FUNCTION_BLOCK "IMAC_MOTOR1_CALL"
TITLE =Function calls for MOTOR1 objects
//Parameter Description for Function MOTOR1 (FB80):
//-------------------------------------------------
//OBJ:     Ascending Object number for MOTOR1 (1...x)
//
//RMOT:    'REMOTE'     Feedback
//                      0 = Local
//                      1 = Remote
//
//RUN:     'RUN'        Feedback
//                      0 = Stopped
//                      1 = Running
//
//FAUL     'EXT. FAULT' Feedback. Function depends on Mode Switch 'ExtFaultNC':
//                      If 'ExtFaultNC' = 0 :       0 = OK,    1 = Fault
//                      If 'ExtFaultNC' = 1 :       0 = Fault, 1 = OK
//
//BLKO:    'BLACKOUT'   Feedback
//                      0 = No Blackout
//                      1 = Blackout
//
//ACOM:    'AUTO' Mode  Command Interface (only active, if 'REMOTE'+'AUTO')
//                      Bit  0       : BlackoutStart
//                      Bit  1       : StandbyActive
//                      Bit  7       : FetchData Command
//                      Bit  8       : Start Command
//                      Bit  9       : Stop  Command
//                      Bit 10       : Failure input from Automatic Function
//                      Bit 11       : Lock 'Start / Stop'
//                      Bit 12       : Emergency Off Command
//
//PCONF:   (leave empty, refers to local instance data in Instance DB)
//
//MSTA:    'START'      Output to Motor
//                      0 = No Command
//                      1 = Start Command
//
//MSTO:    'STOP'       Output to Motor
//                      0 = No Command
//                      1 = Stop Command
//
//ASTAT:   'AUTO' Mode  Status Interface
//                      Bit  8       : Running
//                      Bit  9       : Local
//                      Bit 10       : Manual
//                      Bit 11       : Auto
//                      Bit 12       : Failure
//                      Bit 13       : BlackOut
//                      Bit 14       : Starting
//                      Bit 15       : Restarting
//
//OSSTAT:  OS Status Word
//                      Value = 0    : Undefined
//                      Value = 1    : Running
//                      Value = 2    : Stopped
//                      Value = 3    : Starting
//                      Value = 4    : StandBy
//                      Value = 5    : Blackout
//                      Value + 256  : Local Mode  (Offset Value)
//                      Value + 512  : Manual Mode (Offset Value)
//                      Value + 1024 : Auto Mode   (Offset Value)
//
//OSALARM: OS Alarm Word
//                      Value = 0    : Undefined
//                      Value = 1    : Normal
//                      Value = 2    : External Fault Alarm
//                      Value = 3    : Auto Failure Alarm
//                      Value = 4    : Action Alarm
//                      Value = 5    : Non-Feedback Alarm
//                      Value = 6    : Lock Start / Stop Commands
//                      Value = 7    : Emergency Off
//                      Value = 8    : Blackout
//
//OSCOM:   OS Command Interface
//                      Bit  0       : Start  Command
//                      Bit  1       : Stop   Command
//                      Bit  7       : Reset  Command
//                      Bit  9       : Manual Command
//                      Bit 10       : Auto   Command
AUTHOR : Hottendo
FAMILY : IMAC
VERSION : 0.2


VAR
  motorno_001 : "IMAC_MOTOR1";
  motorno_002 : "IMAC_MOTOR1";
  motorno_003 : "IMAC_MOTOR1";
  motorno_004 : "IMAC_MOTOR1";
  motorno_005 : "IMAC_MOTOR1";
  motorno_006 : "IMAC_MOTOR1";
  motorno_007 : "IMAC_MOTOR1";
  motorno_008 : "IMAC_MOTOR1";
  motorno_009 : "IMAC_MOTOR1";
  motorno_010 : "IMAC_MOTOR1";
  motorno_011 : "IMAC_MOTOR1";
  motorno_012 : "IMAC_MOTOR1";
  motorno_013 : "IMAC_MOTOR1";
  motorno_014 : "IMAC_MOTOR1";
  motorno_015 : "IMAC_MOTOR1";
  motorno_016 : "IMAC_MOTOR1";
  motorno_017 : "IMAC_MOTOR1";
  motorno_018 : "IMAC_MOTOR1";
  motorno_019 : "IMAC_MOTOR1";
  motorno_020 : "IMAC_MOTOR1";
  motorno_021 : "IMAC_MOTOR1";
  motorno_022 : "IMAC_MOTOR1";
  motorno_023 : "IMAC_MOTOR1";
  motorno_024 : "IMAC_MOTOR1";
  motorno_025 : "IMAC_MOTOR1";
  motorno_026 : "IMAC_MOTOR1";
  motorno_027 : "IMAC_MOTOR1";
  motorno_028 : "IMAC_MOTOR1";
  motorno_029 : "IMAC_MOTOR1";
  motorno_030 : "IMAC_MOTOR1";
  motorno_031 : "IMAC_MOTOR1";
  motorno_032 : "IMAC_MOTOR1";
  motorno_033 : "IMAC_MOTOR1";
  motorno_034 : "IMAC_MOTOR1";
  motorno_035 : "IMAC_MOTOR1";
  motorno_036 : "IMAC_MOTOR1";
  motorno_037 : "IMAC_MOTOR1";
  motorno_038 : "IMAC_MOTOR1";
  motorno_039 : "IMAC_MOTOR1";
  motorno_040 : "IMAC_MOTOR1";
  motorno_041 : "IMAC_MOTOR1";
  motorno_042 : "IMAC_MOTOR1";
  motorno_043 : "IMAC_MOTOR1";
  motorno_044 : "IMAC_MOTOR1";
  motorno_045 : "IMAC_MOTOR1";
  motorno_046 : "IMAC_MOTOR1";
  motorno_047 : "IMAC_MOTOR1";
  motorno_048 : "IMAC_MOTOR1";
  motorno_049 : "IMAC_MOTOR1";
  motorno_050 : "IMAC_MOTOR1";
END_VAR
BEGIN
NETWORK
TITLE =MOTOR1 Number 001

      CALL #motorno_001 (
           OBJ                      := 1,
           RMOT                     := E      2.0,
           RUN                      := E      2.1,
           FAUL                     := E      2.2,
           BLKO                     := E      2.3,
           ACOM                     := "IMAC_MOTOR1_I/O".MOTOR1_001_ACOM,
           MSTA                     := A      0.4,
           MSTO                     := A      0.5,
           ASTAT                    := "IMAC_MOTOR1_I/O".MOTOR1_001_ASTAT,
           OSSTAT                   := "IMAC_MOTOR1_I/O".MOTOR1_001_OSSTAT,
           OSALARM                  := "IMAC_MOTOR1_I/O".MOTOR1_001_OSALARM,
           OSCOM                    := "IMAC_MOTOR1_I/O".MOTOR1_001_OSCOM);

NETWORK
TITLE =MOTOR1 Number 002

      CALL #motorno_002 (
           OBJ                      := 2,
           RMOT                     := E      2.4,
           RUN                      := E      2.5,
           FAUL                     := E      2.6,
           BLKO                     := E      2.7,
           ACOM                     := "IMAC_MOTOR1_I/O".MOTOR1_002_ACOM,
           MSTA                     := A      0.6,
           MSTO                     := A      0.7,
           ASTAT                    := "IMAC_MOTOR1_I/O".MOTOR1_002_ASTAT,
           OSSTAT                   := "IMAC_MOTOR1_I/O".MOTOR1_002_OSSTAT,
           OSALARM                  := "IMAC_MOTOR1_I/O".MOTOR1_002_OSALARM,
           OSCOM                    := "IMAC_MOTOR1_I/O".MOTOR1_002_OSCOM);

NETWORK
TITLE =MOTOR1 Number 003

      CALL #motorno_003 (
           OBJ                      := 3,
           RMOT                     := E      3.0,
           RUN                      := E      3.1,
           FAUL                     := E      3.2,
           BLKO                     := E      3.3,
           ACOM                     := "IMAC_MOTOR1_I/O".MOTOR1_003_ACOM,
           MSTA                     := A      1.0,
           MSTO                     := A      1.1,
           ASTAT                    := "IMAC_MOTOR1_I/O".MOTOR1_003_ASTAT,
           OSSTAT                   := "IMAC_MOTOR1_I/O".MOTOR1_003_OSSTAT,
           OSALARM                  := "IMAC_MOTOR1_I/O".MOTOR1_003_OSALARM,
           OSCOM                    := "IMAC_MOTOR1_I/O".MOTOR1_003_OSCOM);

NETWORK
TITLE =MOTOR1 Number 004

      CALL #motorno_004 (
           OBJ                      := 4,
           RMOT                     := E      3.4,
           RUN                      := E      3.5,
           FAUL                     := E      3.6,
           BLKO                     := E      3.7,
           ACOM                     := "IMAC_MOTOR1_I/O".MOTOR1_004_ACOM,
           MSTA                     := A      1.2,
           MSTO                     := A      1.3,
           ASTAT                    := "IMAC_MOTOR1_I/O".MOTOR1_004_ASTAT,
           OSSTAT                   := "IMAC_MOTOR1_I/O".MOTOR1_004_OSSTAT,
           OSALARM                  := "IMAC_MOTOR1_I/O".MOTOR1_004_OSALARM,
           OSCOM                    := "IMAC_MOTOR1_I/O".MOTOR1_004_OSCOM);

NETWORK
TITLE =MOTOR1 Number 005

      CALL #motorno_005 (
           OBJ                      := 5,
           RMOT                     := E      4.0,
           RUN                      := E      4.1,
           FAUL                     := E      4.2,
           BLKO                     := E      4.3,
           ACOM                     := "IMAC_MOTOR1_I/O".MOTOR1_005_ACOM,
           MSTA                     := A      1.4,
           MSTO                     := A      1.5,
           ASTAT                    := "IMAC_MOTOR1_I/O".MOTOR1_005_ASTAT,
           OSSTAT                   := "IMAC_MOTOR1_I/O".MOTOR1_005_OSSTAT,
           OSALARM                  := "IMAC_MOTOR1_I/O".MOTOR1_005_OSALARM,
           OSCOM                    := "IMAC_MOTOR1_I/O".MOTOR1_005_OSCOM);

NETWORK
TITLE =MOTOR1 Number 006

      CALL #motorno_006 (
           OBJ                      := 6,
           RMOT                     := E      4.4,
           RUN                      := E      4.5,
           FAUL                     := E      4.6,
           BLKO                     := E      4.7,
           ACOM                     := "IMAC_MOTOR1_I/O".MOTOR1_006_ACOM,
           MSTA                     := A      1.6,
           MSTO                     := A      1.7,
           ASTAT                    := "IMAC_MOTOR1_I/O".MOTOR1_006_ASTAT,
           OSSTAT                   := "IMAC_MOTOR1_I/O".MOTOR1_006_OSSTAT,
           OSALARM                  := "IMAC_MOTOR1_I/O".MOTOR1_006_OSALARM,
           OSCOM                    := "IMAC_MOTOR1_I/O".MOTOR1_006_OSCOM);

NETWORK
TITLE =MOTOR1 Number 007

//*********** END of function Processing ! *******************************************************************
      BEA   ; // Move this Instruction down to the next Network to add one object !
//************************************************************************************************************

      CALL #motorno_007 (
           OBJ                      := 7,
           ACOM                     := "IMAC_MOTOR1_I/O".MOTOR1_007_ACOM,
           ASTAT                    := "IMAC_MOTOR1_I/O".MOTOR1_007_ASTAT,
           OSSTAT                   := "IMAC_MOTOR1_I/O".MOTOR1_007_OSSTAT,
           OSALARM                  := "IMAC_MOTOR1_I/O".MOTOR1_007_OSALARM,
           OSCOM                    := "IMAC_MOTOR1_I/O".MOTOR1_007_OSCOM);

NETWORK
TITLE =MOTOR1 Number 008

      CALL #motorno_008 (
           OBJ                      := 8,
           ACOM                     := "IMAC_MOTOR1_I/O".MOTOR1_008_ACOM,
           ASTAT                    := "IMAC_MOTOR1_I/O".MOTOR1_008_ASTAT,
           OSSTAT                   := "IMAC_MOTOR1_I/O".MOTOR1_008_OSSTAT,
           OSALARM                  := "IMAC_MOTOR1_I/O".MOTOR1_008_OSALARM,
           OSCOM                    := "IMAC_MOTOR1_I/O".MOTOR1_008_OSCOM);

NETWORK
TITLE =MOTOR1 Number 009

      CALL #motorno_009 (
           OBJ                      := 9,
           ACOM                     := "IMAC_MOTOR1_I/O".MOTOR1_009_ACOM,
           ASTAT                    := "IMAC_MOTOR1_I/O".MOTOR1_009_ASTAT,
           OSSTAT                   := "IMAC_MOTOR1_I/O".MOTOR1_009_OSSTAT,
           OSALARM                  := "IMAC_MOTOR1_I/O".MOTOR1_009_OSALARM,
           OSCOM                    := "IMAC_MOTOR1_I/O".MOTOR1_009_OSCOM);

NETWORK
TITLE =MOTOR1 Number 010

      CALL #motorno_010 (
           OBJ                      := 10,
           ACOM                     := "IMAC_MOTOR1_I/O".MOTOR1_010_ACOM,
           ASTAT                    := "IMAC_MOTOR1_I/O".MOTOR1_010_ASTAT,
           OSSTAT                   := "IMAC_MOTOR1_I/O".MOTOR1_010_OSSTAT,
           OSALARM                  := "IMAC_MOTOR1_I/O".MOTOR1_010_OSALARM,
           OSCOM                    := "IMAC_MOTOR1_I/O".MOTOR1_010_OSCOM);

NETWORK
TITLE =MOTOR1 Number 011

      CALL #motorno_011 (
           OBJ                      := 11,
           ACOM                     := "IMAC_MOTOR1_I/O".MOTOR1_011_ACOM,
           ASTAT                    := "IMAC_MOTOR1_I/O".MOTOR1_011_ASTAT,
           OSSTAT                   := "IMAC_MOTOR1_I/O".MOTOR1_011_OSSTAT,
           OSALARM                  := "IMAC_MOTOR1_I/O".MOTOR1_011_OSALARM,
           OSCOM                    := "IMAC_MOTOR1_I/O".MOTOR1_011_OSCOM);

NETWORK
TITLE =MOTOR1 Number 012

      CALL #motorno_012 (
           OBJ                      := 12,
           ACOM                     := "IMAC_MOTOR1_I/O".MOTOR1_012_ACOM,
           ASTAT                    := "IMAC_MOTOR1_I/O".MOTOR1_012_ASTAT,
           OSSTAT                   := "IMAC_MOTOR1_I/O".MOTOR1_012_OSSTAT,
           OSALARM                  := "IMAC_MOTOR1_I/O".MOTOR1_012_OSALARM,
           OSCOM                    := "IMAC_MOTOR1_I/O".MOTOR1_012_OSCOM);

NETWORK
TITLE =MOTOR1 Number 013

      CALL #motorno_013 (
           OBJ                      := 13,
           ACOM                     := "IMAC_MOTOR1_I/O".MOTOR1_013_ACOM,
           ASTAT                    := "IMAC_MOTOR1_I/O".MOTOR1_013_ASTAT,
           OSSTAT                   := "IMAC_MOTOR1_I/O".MOTOR1_013_OSSTAT,
           OSALARM                  := "IMAC_MOTOR1_I/O".MOTOR1_013_OSALARM,
           OSCOM                    := "IMAC_MOTOR1_I/O".MOTOR1_013_OSCOM);

NETWORK
TITLE =MOTOR1 Number 014

      CALL #motorno_014 (
           OBJ                      := 14,
           ACOM                     := "IMAC_MOTOR1_I/O".MOTOR1_014_ACOM,
           ASTAT                    := "IMAC_MOTOR1_I/O".MOTOR1_014_ASTAT,
           OSSTAT                   := "IMAC_MOTOR1_I/O".MOTOR1_014_OSSTAT,
           OSALARM                  := "IMAC_MOTOR1_I/O".MOTOR1_014_OSALARM,
           OSCOM                    := "IMAC_MOTOR1_I/O".MOTOR1_014_OSCOM);

NETWORK
TITLE =MOTOR1 Number 015

      CALL #motorno_015 (
           OBJ                      := 15,
           ACOM                     := "IMAC_MOTOR1_I/O".MOTOR1_015_ACOM,
           ASTAT                    := "IMAC_MOTOR1_I/O".MOTOR1_015_ASTAT,
           OSSTAT                   := "IMAC_MOTOR1_I/O".MOTOR1_015_OSSTAT,
           OSALARM                  := "IMAC_MOTOR1_I/O".MOTOR1_015_OSALARM,
           OSCOM                    := "IMAC_MOTOR1_I/O".MOTOR1_015_OSCOM);

NETWORK
TITLE =MOTOR1 Number 016

      CALL #motorno_016 (
           OBJ                      := 16,
           ACOM                     := "IMAC_MOTOR1_I/O".MOTOR1_016_ACOM,
           ASTAT                    := "IMAC_MOTOR1_I/O".MOTOR1_016_ASTAT,
           OSSTAT                   := "IMAC_MOTOR1_I/O".MOTOR1_016_OSSTAT,
           OSALARM                  := "IMAC_MOTOR1_I/O".MOTOR1_016_OSALARM,
           OSCOM                    := "IMAC_MOTOR1_I/O".MOTOR1_016_OSCOM);

NETWORK
TITLE =MOTOR1 Number 017

      CALL #motorno_017 (
           OBJ                      := 17,
           ACOM                     := "IMAC_MOTOR1_I/O".MOTOR1_017_ACOM,
           ASTAT                    := "IMAC_MOTOR1_I/O".MOTOR1_017_ASTAT,
           OSSTAT                   := "IMAC_MOTOR1_I/O".MOTOR1_017_OSSTAT,
           OSALARM                  := "IMAC_MOTOR1_I/O".MOTOR1_017_OSALARM,
           OSCOM                    := "IMAC_MOTOR1_I/O".MOTOR1_017_OSCOM);

NETWORK
TITLE =MOTOR1 Number 018

      CALL #motorno_018 (
           OBJ                      := 18,
           ACOM                     := "IMAC_MOTOR1_I/O".MOTOR1_018_ACOM,
           ASTAT                    := "IMAC_MOTOR1_I/O".MOTOR1_018_ASTAT,
           OSSTAT                   := "IMAC_MOTOR1_I/O".MOTOR1_018_OSSTAT,
           OSALARM                  := "IMAC_MOTOR1_I/O".MOTOR1_018_OSALARM,
           OSCOM                    := "IMAC_MOTOR1_I/O".MOTOR1_018_OSCOM);

NETWORK
TITLE =MOTOR1 Number 019

      CALL #motorno_019 (
           OBJ                      := 19,
           ACOM                     := "IMAC_MOTOR1_I/O".MOTOR1_019_ACOM,
           ASTAT                    := "IMAC_MOTOR1_I/O".MOTOR1_019_ASTAT,
           OSSTAT                   := "IMAC_MOTOR1_I/O".MOTOR1_019_OSSTAT,
           OSALARM                  := "IMAC_MOTOR1_I/O".MOTOR1_019_OSALARM,
           OSCOM                    := "IMAC_MOTOR1_I/O".MOTOR1_019_OSCOM);

NETWORK
TITLE =MOTOR1 Number 020

      CALL #motorno_020 (
           OBJ                      := 20,
           ACOM                     := "IMAC_MOTOR1_I/O".MOTOR1_020_ACOM,
           ASTAT                    := "IMAC_MOTOR1_I/O".MOTOR1_020_ASTAT,
           OSSTAT                   := "IMAC_MOTOR1_I/O".MOTOR1_020_OSSTAT,
           OSALARM                  := "IMAC_MOTOR1_I/O".MOTOR1_020_OSALARM,
           OSCOM                    := "IMAC_MOTOR1_I/O".MOTOR1_020_OSCOM);

NETWORK
TITLE =MOTOR1 Number 021

      CALL #motorno_021 (
           OBJ                      := 21,
           ACOM                     := "IMAC_MOTOR1_I/O".MOTOR1_021_ACOM,
           ASTAT                    := "IMAC_MOTOR1_I/O".MOTOR1_021_ASTAT,
           OSSTAT                   := "IMAC_MOTOR1_I/O".MOTOR1_021_OSSTAT,
           OSALARM                  := "IMAC_MOTOR1_I/O".MOTOR1_021_OSALARM,
           OSCOM                    := "IMAC_MOTOR1_I/O".MOTOR1_021_OSCOM);

NETWORK
TITLE =MOTOR1 Number 022

      CALL #motorno_022 (
           OBJ                      := 22,
           ACOM                     := "IMAC_MOTOR1_I/O".MOTOR1_022_ACOM,
           ASTAT                    := "IMAC_MOTOR1_I/O".MOTOR1_022_ASTAT,
           OSSTAT                   := "IMAC_MOTOR1_I/O".MOTOR1_022_OSSTAT,
           OSALARM                  := "IMAC_MOTOR1_I/O".MOTOR1_022_OSALARM,
           OSCOM                    := "IMAC_MOTOR1_I/O".MOTOR1_003_OSCOM);

NETWORK
TITLE =MOTOR1 Number 023

      CALL #motorno_023 (
           OBJ                      := 23,
           ACOM                     := "IMAC_MOTOR1_I/O".MOTOR1_023_ACOM,
           ASTAT                    := "IMAC_MOTOR1_I/O".MOTOR1_023_ASTAT,
           OSSTAT                   := "IMAC_MOTOR1_I/O".MOTOR1_023_OSSTAT,
           OSALARM                  := "IMAC_MOTOR1_I/O".MOTOR1_023_OSALARM,
           OSCOM                    := "IMAC_MOTOR1_I/O".MOTOR1_023_OSCOM);

NETWORK
TITLE =MOTOR1 Number 024

      CALL #motorno_024 (
           OBJ                      := 24,
           ACOM                     := "IMAC_MOTOR1_I/O".MOTOR1_024_ACOM,
           ASTAT                    := "IMAC_MOTOR1_I/O".MOTOR1_024_ASTAT,
           OSSTAT                   := "IMAC_MOTOR1_I/O".MOTOR1_024_OSSTAT,
           OSALARM                  := "IMAC_MOTOR1_I/O".MOTOR1_024_OSALARM,
           OSCOM                    := "IMAC_MOTOR1_I/O".MOTOR1_024_OSCOM);

NETWORK
TITLE =MOTOR1 Number 025

      CALL #motorno_025 (
           OBJ                      := 25,
           ACOM                     := "IMAC_MOTOR1_I/O".MOTOR1_025_ACOM,
           ASTAT                    := "IMAC_MOTOR1_I/O".MOTOR1_025_ASTAT,
           OSSTAT                   := "IMAC_MOTOR1_I/O".MOTOR1_025_OSSTAT,
           OSALARM                  := "IMAC_MOTOR1_I/O".MOTOR1_025_OSALARM,
           OSCOM                    := "IMAC_MOTOR1_I/O".MOTOR1_025_OSCOM);

NETWORK
TITLE =MOTOR1 Number 026

      CALL #motorno_026 (
           OBJ                      := 26,
           ACOM                     := "IMAC_MOTOR1_I/O".MOTOR1_026_ACOM,
           ASTAT                    := "IMAC_MOTOR1_I/O".MOTOR1_026_ASTAT,
           OSSTAT                   := "IMAC_MOTOR1_I/O".MOTOR1_026_OSSTAT,
           OSALARM                  := "IMAC_MOTOR1_I/O".MOTOR1_026_OSALARM,
           OSCOM                    := "IMAC_MOTOR1_I/O".MOTOR1_026_OSCOM);

NETWORK
TITLE =MOTOR1 Number 027

      CALL #motorno_027 (
           OBJ                      := 27,
           ACOM                     := "IMAC_MOTOR1_I/O".MOTOR1_027_ACOM,
           ASTAT                    := "IMAC_MOTOR1_I/O".MOTOR1_027_ASTAT,
           OSSTAT                   := "IMAC_MOTOR1_I/O".MOTOR1_027_OSSTAT,
           OSALARM                  := "IMAC_MOTOR1_I/O".MOTOR1_027_OSALARM,
           OSCOM                    := "IMAC_MOTOR1_I/O".MOTOR1_027_OSCOM);

NETWORK
TITLE =MOTOR1 Number 028

      CALL #motorno_028 (
           OBJ                      := 28,
           ACOM                     := "IMAC_MOTOR1_I/O".MOTOR1_028_ACOM,
           ASTAT                    := "IMAC_MOTOR1_I/O".MOTOR1_028_ASTAT,
           OSSTAT                   := "IMAC_MOTOR1_I/O".MOTOR1_028_OSSTAT,
           OSALARM                  := "IMAC_MOTOR1_I/O".MOTOR1_028_OSALARM,
           OSCOM                    := "IMAC_MOTOR1_I/O".MOTOR1_028_OSCOM);

NETWORK
TITLE =MOTOR1 Number 029

      CALL #motorno_029 (
           OBJ                      := 29,
           ACOM                     := "IMAC_MOTOR1_I/O".MOTOR1_029_ACOM,
           ASTAT                    := "IMAC_MOTOR1_I/O".MOTOR1_029_ASTAT,
           OSSTAT                   := "IMAC_MOTOR1_I/O".MOTOR1_029_OSSTAT,
           OSALARM                  := "IMAC_MOTOR1_I/O".MOTOR1_029_OSALARM,
           OSCOM                    := "IMAC_MOTOR1_I/O".MOTOR1_029_OSCOM);

NETWORK
TITLE =MOTOR1 Number 030

      CALL #motorno_030 (
           OBJ                      := 30,
           ACOM                     := "IMAC_MOTOR1_I/O".MOTOR1_030_ACOM,
           ASTAT                    := "IMAC_MOTOR1_I/O".MOTOR1_030_ASTAT,
           OSSTAT                   := "IMAC_MOTOR1_I/O".MOTOR1_030_OSSTAT,
           OSALARM                  := "IMAC_MOTOR1_I/O".MOTOR1_030_OSALARM,
           OSCOM                    := "IMAC_MOTOR1_I/O".MOTOR1_030_OSCOM);

NETWORK
TITLE =MOTOR1 Number 031

      CALL #motorno_031 (
           OBJ                      := 31,
           ACOM                     := "IMAC_MOTOR1_I/O".MOTOR1_031_ACOM,
           ASTAT                    := "IMAC_MOTOR1_I/O".MOTOR1_031_ASTAT,
           OSSTAT                   := "IMAC_MOTOR1_I/O".MOTOR1_031_OSSTAT,
           OSALARM                  := "IMAC_MOTOR1_I/O".MOTOR1_031_OSALARM,
           OSCOM                    := "IMAC_MOTOR1_I/O".MOTOR1_031_OSCOM);

NETWORK
TITLE =MOTOR1 Number 032

      CALL #motorno_032 (
           OBJ                      := 32,
           ACOM                     := "IMAC_MOTOR1_I/O".MOTOR1_032_ACOM,
           ASTAT                    := "IMAC_MOTOR1_I/O".MOTOR1_032_ASTAT,
           OSSTAT                   := "IMAC_MOTOR1_I/O".MOTOR1_032_OSSTAT,
           OSALARM                  := "IMAC_MOTOR1_I/O".MOTOR1_032_OSALARM,
           OSCOM                    := "IMAC_MOTOR1_I/O".MOTOR1_032_OSCOM);

NETWORK
TITLE =MOTOR1 Number 033

      CALL #motorno_033 (
           OBJ                      := 33,
           ACOM                     := "IMAC_MOTOR1_I/O".MOTOR1_033_ACOM,
           ASTAT                    := "IMAC_MOTOR1_I/O".MOTOR1_033_ASTAT,
           OSSTAT                   := "IMAC_MOTOR1_I/O".MOTOR1_033_OSSTAT,
           OSALARM                  := "IMAC_MOTOR1_I/O".MOTOR1_033_OSALARM,
           OSCOM                    := "IMAC_MOTOR1_I/O".MOTOR1_033_OSCOM);

NETWORK
TITLE =MOTOR1 Number 034

      CALL #motorno_034 (
           OBJ                      := 34,
           ACOM                     := "IMAC_MOTOR1_I/O".MOTOR1_034_ACOM,
           ASTAT                    := "IMAC_MOTOR1_I/O".MOTOR1_034_ASTAT,
           OSSTAT                   := "IMAC_MOTOR1_I/O".MOTOR1_034_OSSTAT,
           OSALARM                  := "IMAC_MOTOR1_I/O".MOTOR1_034_OSALARM,
           OSCOM                    := "IMAC_MOTOR1_I/O".MOTOR1_034_OSCOM);

NETWORK
TITLE =MOTOR1 Number 035

      CALL #motorno_035 (
           OBJ                      := 35,
           ACOM                     := "IMAC_MOTOR1_I/O".MOTOR1_035_ACOM,
           ASTAT                    := "IMAC_MOTOR1_I/O".MOTOR1_035_ASTAT,
           OSSTAT                   := "IMAC_MOTOR1_I/O".MOTOR1_035_OSSTAT,
           OSALARM                  := "IMAC_MOTOR1_I/O".MOTOR1_035_OSALARM,
           OSCOM                    := "IMAC_MOTOR1_I/O".MOTOR1_035_OSCOM);

NETWORK
TITLE =MOTOR1 Number 036

      CALL #motorno_036 (
           OBJ                      := 36,
           ACOM                     := "IMAC_MOTOR1_I/O".MOTOR1_036_ACOM,
           ASTAT                    := "IMAC_MOTOR1_I/O".MOTOR1_036_ASTAT,
           OSSTAT                   := "IMAC_MOTOR1_I/O".MOTOR1_036_OSSTAT,
           OSALARM                  := "IMAC_MOTOR1_I/O".MOTOR1_036_OSALARM,
           OSCOM                    := "IMAC_MOTOR1_I/O".MOTOR1_036_OSCOM);

NETWORK
TITLE =MOTOR1 Number 037

      CALL #motorno_037 (
           OBJ                      := 37,
           ACOM                     := "IMAC_MOTOR1_I/O".MOTOR1_037_ACOM,
           ASTAT                    := "IMAC_MOTOR1_I/O".MOTOR1_037_ASTAT,
           OSSTAT                   := "IMAC_MOTOR1_I/O".MOTOR1_037_OSSTAT,
           OSALARM                  := "IMAC_MOTOR1_I/O".MOTOR1_037_OSALARM,
           OSCOM                    := "IMAC_MOTOR1_I/O".MOTOR1_037_OSCOM);

NETWORK
TITLE =MOTOR1 Number 038

      CALL #motorno_038 (
           OBJ                      := 38,
           ACOM                     := "IMAC_MOTOR1_I/O".MOTOR1_038_ACOM,
           ASTAT                    := "IMAC_MOTOR1_I/O".MOTOR1_038_ASTAT,
           OSSTAT                   := "IMAC_MOTOR1_I/O".MOTOR1_038_OSSTAT,
           OSALARM                  := "IMAC_MOTOR1_I/O".MOTOR1_038_OSALARM,
           OSCOM                    := "IMAC_MOTOR1_I/O".MOTOR1_038_OSCOM);

NETWORK
TITLE =MOTOR1 Number 039

      CALL #motorno_039 (
           OBJ                      := 39,
           ACOM                     := "IMAC_MOTOR1_I/O".MOTOR1_039_ACOM,
           ASTAT                    := "IMAC_MOTOR1_I/O".MOTOR1_039_ASTAT,
           OSSTAT                   := "IMAC_MOTOR1_I/O".MOTOR1_039_OSSTAT,
           OSALARM                  := "IMAC_MOTOR1_I/O".MOTOR1_039_OSALARM,
           OSCOM                    := "IMAC_MOTOR1_I/O".MOTOR1_039_OSCOM);

NETWORK
TITLE =MOTOR1 Number 040

      CALL #motorno_040 (
           OBJ                      := 40,
           ACOM                     := "IMAC_MOTOR1_I/O".MOTOR1_040_ACOM,
           ASTAT                    := "IMAC_MOTOR1_I/O".MOTOR1_040_ASTAT,
           OSSTAT                   := "IMAC_MOTOR1_I/O".MOTOR1_040_OSSTAT,
           OSALARM                  := "IMAC_MOTOR1_I/O".MOTOR1_040_OSALARM,
           OSCOM                    := "IMAC_MOTOR1_I/O".MOTOR1_040_OSCOM);

NETWORK
TITLE =MOTOR1 Number 041

      CALL #motorno_041 (
           OBJ                      := 41,
           ACOM                     := "IMAC_MOTOR1_I/O".MOTOR1_041_ACOM,
           ASTAT                    := "IMAC_MOTOR1_I/O".MOTOR1_041_ASTAT,
           OSSTAT                   := "IMAC_MOTOR1_I/O".MOTOR1_041_OSSTAT,
           OSALARM                  := "IMAC_MOTOR1_I/O".MOTOR1_041_OSALARM,
           OSCOM                    := "IMAC_MOTOR1_I/O".MOTOR1_041_OSCOM);

NETWORK
TITLE =MOTOR1 Number 042

      CALL #motorno_042 (
           OBJ                      := 42,
           ACOM                     := "IMAC_MOTOR1_I/O".MOTOR1_042_ACOM,
           ASTAT                    := "IMAC_MOTOR1_I/O".MOTOR1_042_ASTAT,
           OSSTAT                   := "IMAC_MOTOR1_I/O".MOTOR1_042_OSSTAT,
           OSALARM                  := "IMAC_MOTOR1_I/O".MOTOR1_042_OSALARM,
           OSCOM                    := "IMAC_MOTOR1_I/O".MOTOR1_042_OSCOM);

NETWORK
TITLE =MOTOR1 Number 043

      CALL #motorno_043 (
           OBJ                      := 43,
           ACOM                     := "IMAC_MOTOR1_I/O".MOTOR1_043_ACOM,
           ASTAT                    := "IMAC_MOTOR1_I/O".MOTOR1_043_ASTAT,
           OSSTAT                   := "IMAC_MOTOR1_I/O".MOTOR1_043_OSSTAT,
           OSALARM                  := "IMAC_MOTOR1_I/O".MOTOR1_043_OSALARM,
           OSCOM                    := "IMAC_MOTOR1_I/O".MOTOR1_043_OSCOM);

NETWORK
TITLE =MOTOR1 Number 044

      CALL #motorno_044 (
           OBJ                      := 44,
           ACOM                     := "IMAC_MOTOR1_I/O".MOTOR1_044_ACOM,
           ASTAT                    := "IMAC_MOTOR1_I/O".MOTOR1_044_ASTAT,
           OSSTAT                   := "IMAC_MOTOR1_I/O".MOTOR1_044_OSSTAT,
           OSALARM                  := "IMAC_MOTOR1_I/O".MOTOR1_044_OSALARM,
           OSCOM                    := "IMAC_MOTOR1_I/O".MOTOR1_044_OSCOM);

NETWORK
TITLE =MOTOR1 Number 045

      CALL #motorno_045 (
           OBJ                      := 45,
           ACOM                     := "IMAC_MOTOR1_I/O".MOTOR1_045_ACOM,
           ASTAT                    := "IMAC_MOTOR1_I/O".MOTOR1_045_ASTAT,
           OSSTAT                   := "IMAC_MOTOR1_I/O".MOTOR1_045_OSSTAT,
           OSALARM                  := "IMAC_MOTOR1_I/O".MOTOR1_045_OSALARM,
           OSCOM                    := "IMAC_MOTOR1_I/O".MOTOR1_045_OSCOM);

NETWORK
TITLE =MOTOR1 Number 046

      CALL #motorno_046 (
           OBJ                      := 46,
           ACOM                     := "IMAC_MOTOR1_I/O".MOTOR1_046_ACOM,
           ASTAT                    := "IMAC_MOTOR1_I/O".MOTOR1_046_ASTAT,
           OSSTAT                   := "IMAC_MOTOR1_I/O".MOTOR1_046_OSSTAT,
           OSALARM                  := "IMAC_MOTOR1_I/O".MOTOR1_046_OSALARM,
           OSCOM                    := "IMAC_MOTOR1_I/O".MOTOR1_046_OSCOM);

NETWORK
TITLE =MOTOR1 Number 047

      CALL #motorno_047 (
           OBJ                      := 47,
           ACOM                     := "IMAC_MOTOR1_I/O".MOTOR1_047_ACOM,
           ASTAT                    := "IMAC_MOTOR1_I/O".MOTOR1_047_ASTAT,
           OSSTAT                   := "IMAC_MOTOR1_I/O".MOTOR1_047_OSSTAT,
           OSALARM                  := "IMAC_MOTOR1_I/O".MOTOR1_047_OSALARM,
           OSCOM                    := "IMAC_MOTOR1_I/O".MOTOR1_047_OSCOM);

NETWORK
TITLE =MOTOR1 Number 048

      CALL #motorno_048 (
           OBJ                      := 48,
           ACOM                     := "IMAC_MOTOR1_I/O".MOTOR1_048_ACOM,
           ASTAT                    := "IMAC_MOTOR1_I/O".MOTOR1_048_ASTAT,
           OSSTAT                   := "IMAC_MOTOR1_I/O".MOTOR1_048_OSSTAT,
           OSALARM                  := "IMAC_MOTOR1_I/O".MOTOR1_048_OSALARM,
           OSCOM                    := "IMAC_MOTOR1_I/O".MOTOR1_048_OSCOM);

NETWORK
TITLE =MOTOR1 Number 049

      CALL #motorno_049 (
           OBJ                      := 49,
           ACOM                     := "IMAC_MOTOR1_I/O".MOTOR1_049_ACOM,
           ASTAT                    := "IMAC_MOTOR1_I/O".MOTOR1_049_ASTAT,
           OSSTAT                   := "IMAC_MOTOR1_I/O".MOTOR1_049_OSSTAT,
           OSALARM                  := "IMAC_MOTOR1_I/O".MOTOR1_049_OSALARM,
           OSCOM                    := "IMAC_MOTOR1_I/O".MOTOR1_049_OSCOM);

NETWORK
TITLE =MOTOR1 Number 050

      CALL #motorno_050 (
           OBJ                      := 50,
           ACOM                     := "IMAC_MOTOR1_I/O".MOTOR1_050_ACOM,
           ASTAT                    := "IMAC_MOTOR1_I/O".MOTOR1_050_ASTAT,
           OSSTAT                   := "IMAC_MOTOR1_I/O".MOTOR1_050_OSSTAT,
           OSALARM                  := "IMAC_MOTOR1_I/O".MOTOR1_050_OSALARM,
           OSCOM                    := "IMAC_MOTOR1_I/O".MOTOR1_050_OSCOM);

END_FUNCTION_BLOCK

